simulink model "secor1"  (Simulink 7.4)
settings: Solver=ode45  StartTime=0.0  StopTime=20  MaxStep=0.02  RelTol=1e-3  AbsTol=1e-3
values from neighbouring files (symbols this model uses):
  omega = 1    [eksper.m]    (also in eksper_sim_step.m; ZRS2_primer_3_9_a.m = linspace(0.25,0.60,100); ZRS2_sl_2_13.m)
undefined symbols (not defined in the file or in its folder): zeta

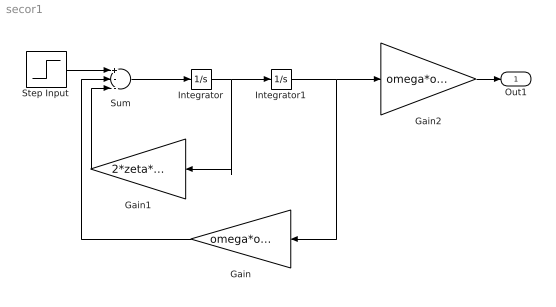
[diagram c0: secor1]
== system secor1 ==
  Gain : Gain  Gain=omega*omega  ParameterDataType=sfix(16)  ParameterScaling=2^0  OutDataType=sfix(16)  OutScaling=2^0
  Gain1 : Gain  Gain=2*zeta*omega  ParameterDataType=sfix(16)  ParameterScaling=2^0  OutDataType=sfix(16)  OutScaling=2^0
  Gain2 : Gain  Gain=omega*omega  ParameterDataType=sfix(16)  ParameterScaling=2^0  OutDataType=sfix(16)  OutScaling=2^0
  Integrator : Integrator
  Integrator1 : Integrator
  Step Input : Step  Time=0  SampleTime=0
  Sum : Sum  Inputs=+--  OutDataType=sfix(16)  OutScaling=2^0
  Out1 : Outport  OutDataType=sfix(16)  OutScaling=2^0
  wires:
  Sum/1 -> Integrator/1
  Step Input/1 -> Sum/1
  Integrator/1 -> Integrator1/1, Gain1/1
  Gain1/1 -> Sum/3
  Gain/1 -> Sum/2
  Integrator1/1 -> Gain/1, Gain2/1
  Gain2/1 -> Out1/1
